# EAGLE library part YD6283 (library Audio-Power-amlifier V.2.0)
YD6283 is an audio power IC with built-in two channels developed for portable radio cassette tape recorder. Because of the parts reduction and SIP (Single In line Package), space merit is remarkable. Thermal shut down protection circuit is built in.
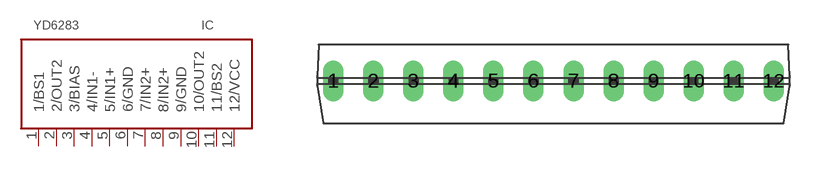
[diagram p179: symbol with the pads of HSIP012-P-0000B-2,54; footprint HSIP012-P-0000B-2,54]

Designator prefix IC

## YD6283  [HSIP012-P-0000B-2,54]
1  1/BS1  in
2  2/OUT2  out
3  3/BIAS  out
4  4/IN1-  in
5  5/IN1+  in
6  6/GND  pwr
7  7/IN2+  in
8  8/IN2+  in
9  9/GND  pwr
10  10/OUT2  out
11  11/BS2  out
12  12/VCC  pwr

## Footprint HSIP012-P-0000B-2,54 (pad centres in mm)
drill 0.8 long: 1 -13.97,0; 2 -11.43,0; 3 -8.89,0; 4 -6.35,0; 5 -3.81,0; 6 -1.27,0; 7 1.27,0; 8 3.81,0; 9 6.35,0; 10 8.89,0; 11 11.43,0; 12 13.97,0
